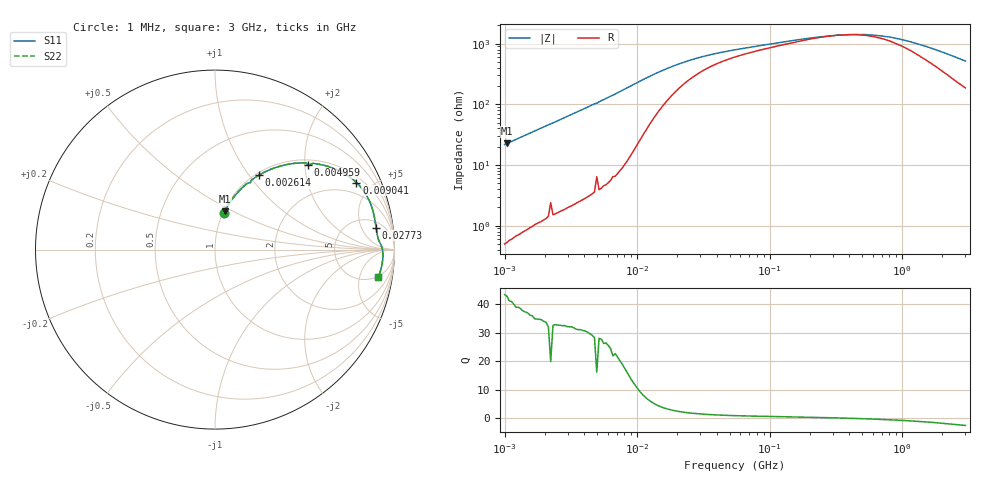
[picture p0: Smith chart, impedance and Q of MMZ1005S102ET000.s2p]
! S-parameter Generated by TDK Corporation
! Copyright(C) 2016 TDK Corporation.
! All Rights Reserved.
! TDK P/N: MMZ1005S102ET000 (Chip Beads)
! Property: |Z|=1000¶ at 100MHz
! Size(LxWxT): 1x0.5x0.5mm, 0.039x0.02x0.02inches
! Model Type: s2p (Touchstone File Format Version 1.0)
! Frequency: DC=Yes Start=1MHz Stop=3000MHz 202points Log-sweep
! Note: This model was converted from impedance.
! Model Generated on May. 16, 2016
! Hash(MD5):
! Port Assignments:
!  1 ---@@@--- 2
! Applicable Conditions:
!  Temperature = 25 degC
!  DC Bias Current = 0 A
!  Small Signal Operation
! Terms and conditions regarding TDK Simulation Models
! (1)This simulation model is being provided solely for informational purposes. Please refer to the specifications of the products in terms of detailed characteristics of such products.
! (2)In no event shall TDK Corporation of any of its subsidiaries be liable for any loss or damage arising, directly or indirectly,
!  From any information contained in this simulation model, including, but not limited to loss or damages arising from any inaccuracies, omissions or errors in connection with such information.
! (3)Any and all copyrights on this simulation model are owned by TDK Corporation.
!  Duplication or redistribution of this simulation model without prior written permission from TDK Corporation is prohibited.
! (4)This simulation model is subject to any modification or change without any prior notice.
! (5)Neither TDK Corporation nor any of its subsidiaries shall make any warranty, express or implied,
!  Including but not limited to the correctness, implied warranties of merchantability and fitness for a particular purpose with respect to this simulation models.
! (6)The use of this simulation model shall be deemed to have consented to the terms and conditions hereof.
# MHz S MA R 50
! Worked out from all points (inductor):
!   201 points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, 1 MHz to 3 GHz, reference 50 ohm
!   read as one part in series: L = 3.45 uH near 1.041 MHz
!   highest Q = 42.9 at 1.041 MHz (marker M1), where L = 3.46 uH
!   self-resonance near 358.9 MHz
!   S11 on the Smith chart (normalised r, x): 1 MHz: 1.01, +0.43; 2.614 MHz: 1.03, +1.11; 4.959 MHz: 1.13, +2.07; 9.041 MHz: 1.30, +4.05; 27.73 MHz: 7, +10; 3 GHz: 5, -10
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1  0.2113 76.5  0.9726 -12.2  0.9726 -12.2  0.2113 76.5
1.040844  0.2195 76.0  0.9705 -12.7  0.9705 -12.7  0.2195 76.0
1.682724  0.3376 68.6  0.9317 -19.7  0.9317 -19.7  0.3376 68.6
2.613693  0.4804 59.6  0.8625 -28.7  0.8625 -28.7  0.4804 59.6
3.900413  0.6285 49.2  0.7577 -38.9  0.7577 -38.9  0.6285 49.2
4.764734  0.701 43.5  0.6889 -44.5  0.6889 -44.5  0.701 43.5
4.959344  0.6994 42.2  0.6729 -44.3  0.6729 -44.3  0.6994 42.2
5.161903  0.7273 41.3  0.6609 -46.6  0.6609 -46.6  0.7273 41.3
6.305767  0.7904 35.5  0.5812 -52.2  0.5812 -52.2  0.7904 35.5
9.040831  0.8721 25.4  0.4293 -60.4  0.4293 -60.4  0.8721 25.4
11.49534  0.8973 19.5  0.3373 -62.8  0.3373 -62.8  0.8973 19.5
14.61624  0.9054 15.0  0.2652 -61.8  0.2652 -61.8  0.9054 15.0
20.13356  0.9064 10.6  0.1997 -56.9  0.1997 -56.9  0.9064 10.6
27.73354  0.9063 7.7  0.159 -50.1  0.159 -50.1  0.9063 7.7
54.77226  0.9098 4.3  0.1148 -36.1  0.1148 -36.1  0.9098 4.3
213.6344  0.9284 1.1  0.07394 -13.8  0.07394 -13.8  0.9284 1.1
439.1493  0.9345 -0.5  0.0659 6.4  0.0659 6.4  0.9345 -0.5
581.181  0.9357 -1.1  0.06714 16.1  0.06714 16.1  0.9357 -1.1
800.5644  0.9366 -2.1  0.07265 28.2  0.07265 28.2  0.9366 -2.1
1059.487  0.9363 -3.1  0.08271 38.1  0.08271 38.1  0.9363 -3.1
1519.029  0.9346 -4.8  0.1039 48.7  0.1039 48.7  0.9346 -4.8
3000  0.922 -9.6  0.1782 59.3  0.1782 59.3  0.922 -9.6
